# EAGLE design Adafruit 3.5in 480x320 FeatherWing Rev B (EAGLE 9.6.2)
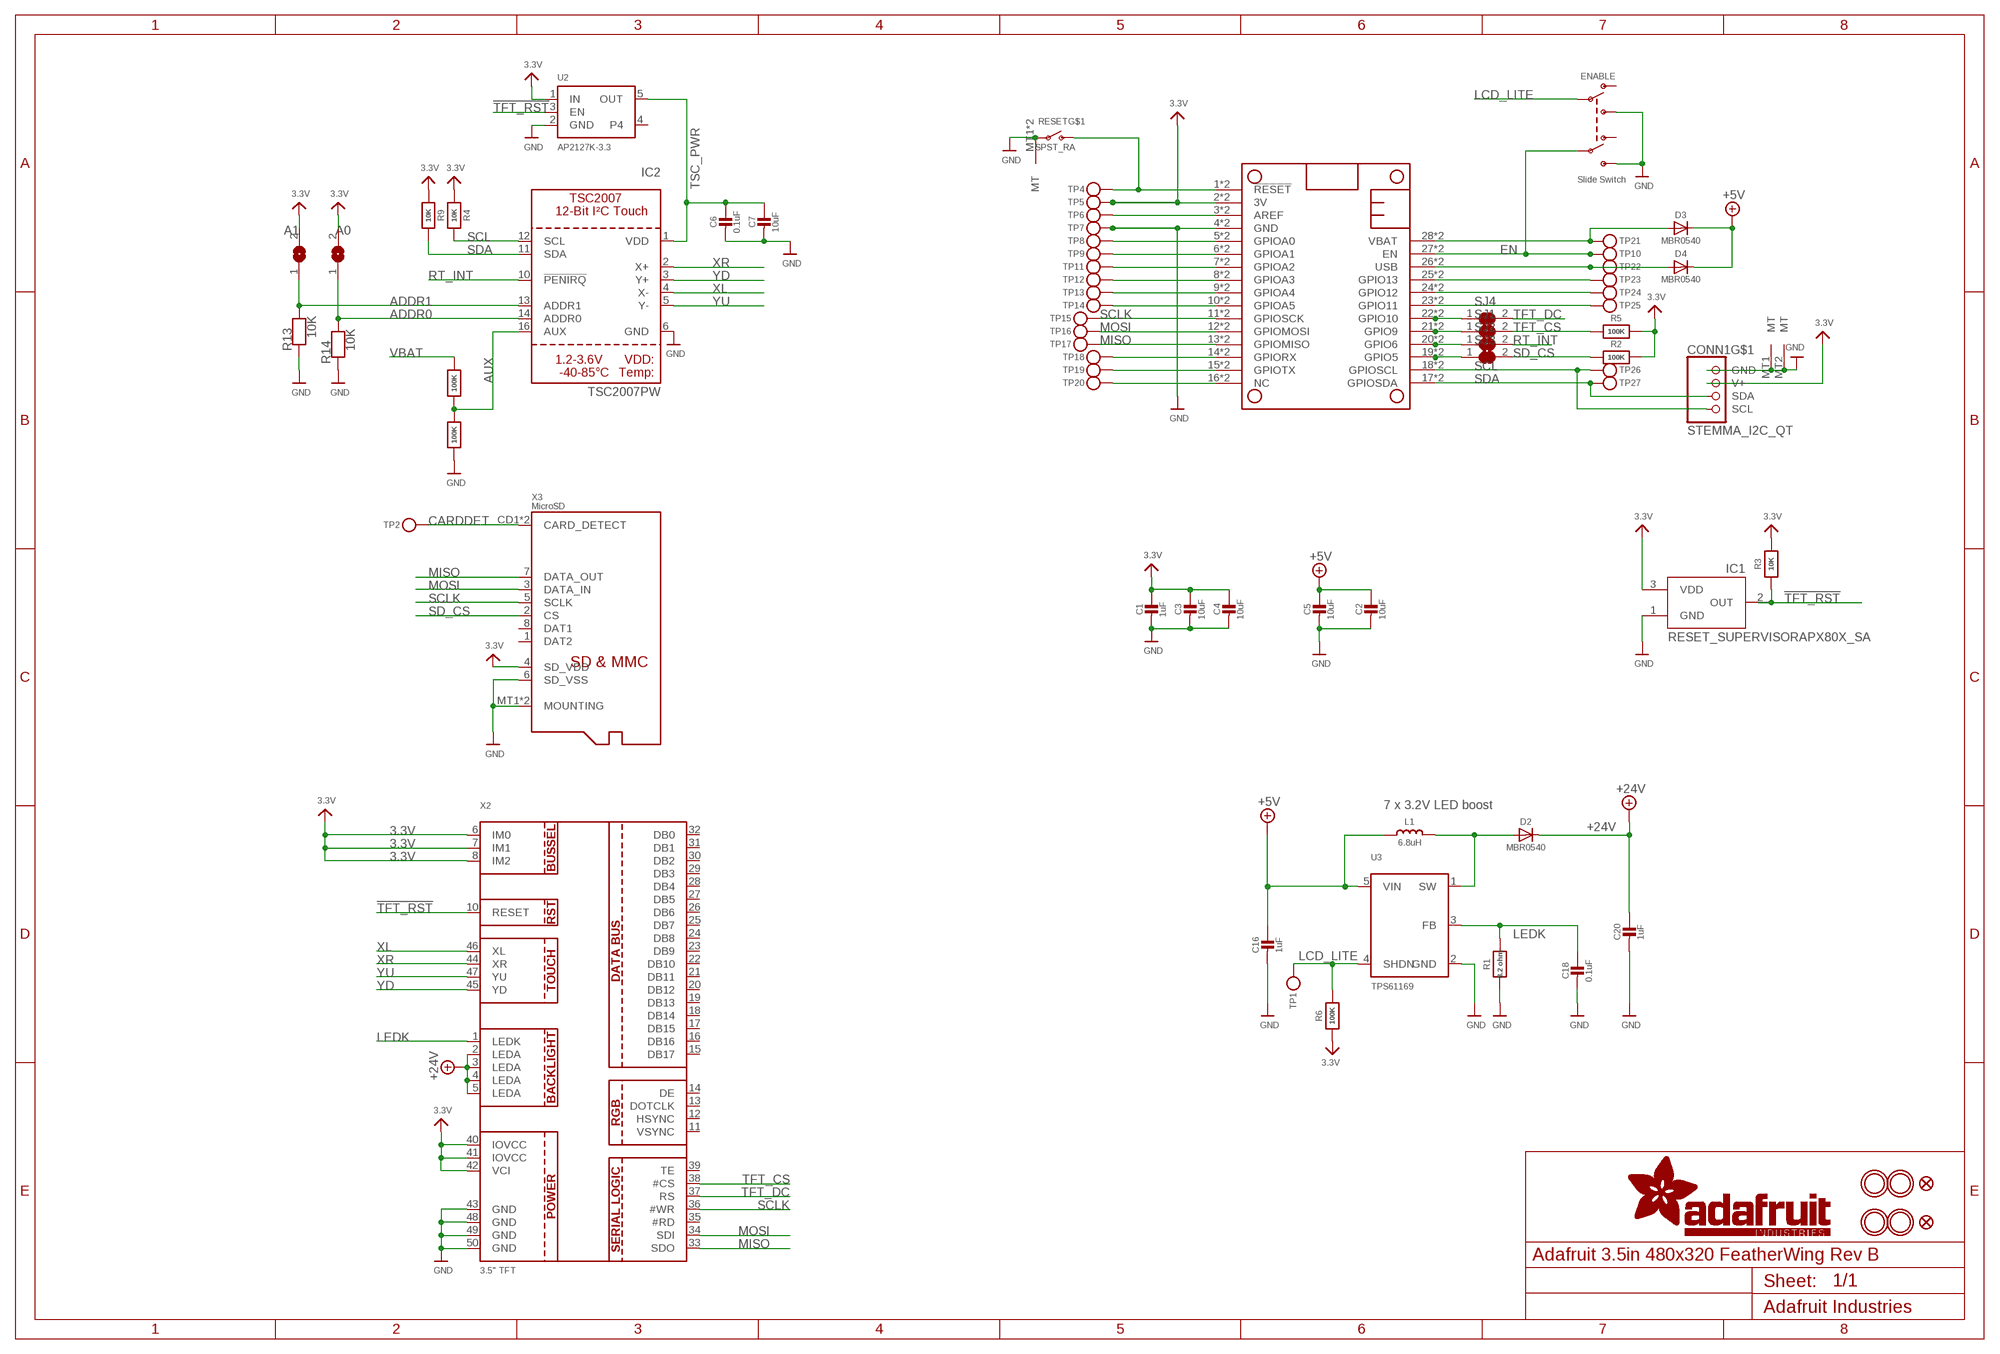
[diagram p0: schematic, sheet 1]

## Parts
C1  1uF  CAP_CERAMIC0805-NOOUTLINE  [0805-NO]
C2  10uF  CAP_CERAMIC0805-NOOUTLINE  [0805-NO]
C3  10uF  CAP_CERAMIC0805-NOOUTLINE  [0805-NO]
C4  10uF  CAP_CERAMIC0805-NOOUTLINE  [0805-NO]
C5  10uF  CAP_CERAMIC0805-NOOUTLINE  [0805-NO]
C6  0.1uF  CAP_CERAMIC0603_NO  [0603-NO]
C7  10uF  CAP_CERAMIC0805-NOOUTLINE  [0805-NO]
C16  1uF  CAP_CERAMIC0805-NOOUTLINE  [0805-NO]
C18  0.1uF  CAP_CERAMIC0603_NO  [0603-NO]
C20  1uF  CAP_CERAMIC0805-NOOUTLINE  [0805-NO]
CONN1  STEMMA_I2C_QT  [JST_SH4]
D2  MBR0540  DIODESOD-123  [SOD-123]
D3  MBR0540  DIODESOD-123  [SOD-123]
D4  MBR0540  DIODESOD-123  [SOD-123]
ENABLE  Slide Switch  SWITCH_DPDTEG1390  [EG1390]
IC1  RESET_SUPERVISORAPX80X_SA  [SOT23-WIDE]
IC2  TSC2007PW  [TSSOP16]
ICSP_CLK1  A1  SOLDERJUMPER  [SOLDERJUMPER_ARROW_NOPASTE]
ICSP_CLK2  A0  SOLDERJUMPER  [SOLDERJUMPER_ARROW_NOPASTE]
L1  6.8uH  INDUCTORNR5040  [INDUCTOR_5X5MM_NR5040_NOTHERMALS]
MS2  FEATHERWING_SMTDUAL  [FEATHERWING_SMT2]
R1  8.2 ohm  RESISTOR_0603_NOOUT  [0603-NO]
R2  100K  RESISTOR_0603_NOOUT  [0603-NO]
R3  10K  RESISTOR_0603_NOOUT  [0603-NO]
R4  10K  RESISTOR_0603_NOOUT  [0603-NO]
R5  100K  RESISTOR_0603_NOOUT  [0603-NO]
R6  100K  RESISTOR_0603_NOOUT  [0603-NO]
R9  10K  RESISTOR_0603_NOOUT  [0603-NO]
R10  100K  RESISTOR_0603_NOOUT  [0603-NO]
R11  100K  RESISTOR_0603_NOOUT  [0603-NO]
R13  10K  RESISTOR_0603_NOOUT  [0603-NO]
R14  10K  RESISTOR_0603_NOOUT  [0603-NO]
RESET  SPST_RA  SWITCH_SPST_MNT_TACT_RA  [SPST_TACTILE_RA]
SJ1  SOLDERJUMPER_CLOSED  [SOLDERJUMPER_CLOSEDWIRE]
SJ2  SOLDERJUMPER_CLOSED  [SOLDERJUMPER_CLOSEDWIRE]
SJ3  SOLDERJUMPER_CLOSED  [SOLDERJUMPER_CLOSEDWIRE]
SJ4  SOLDERJUMPER_CLOSED  [SOLDERJUMPER_CLOSEDWIRE]
TP1  TESTPOINTPAD2MM  [TESTPOINT_PAD_2MM]
TP2  TESTPOINTPAD2MM  [TESTPOINT_PAD_2MM]
TP4  TESTPOINTPAD2MM  [TESTPOINT_PAD_2MM]
TP5  TESTPOINTPAD2MM  [TESTPOINT_PAD_2MM]
TP6  TESTPOINTPAD2MM  [TESTPOINT_PAD_2MM]
TP7  TESTPOINTPAD2MM  [TESTPOINT_PAD_2MM]
TP8  TESTPOINTPAD2MM  [TESTPOINT_PAD_2MM]
TP9  TESTPOINTPAD2MM  [TESTPOINT_PAD_2MM]
TP10  TESTPOINTPAD2MM  [TESTPOINT_PAD_2MM]
TP11  TESTPOINTPAD2MM  [TESTPOINT_PAD_2MM]
TP12  TESTPOINTPAD2MM  [TESTPOINT_PAD_2MM]
TP13  TESTPOINTPAD2MM  [TESTPOINT_PAD_2MM]
TP14  TESTPOINTPAD2MM  [TESTPOINT_PAD_2MM]
TP15  TESTPOINTPAD2MM  [TESTPOINT_PAD_2MM]
TP16  TESTPOINTPAD2MM  [TESTPOINT_PAD_2MM]
TP17  TESTPOINTPAD2MM  [TESTPOINT_PAD_2MM]
TP18  TESTPOINTPAD2MM  [TESTPOINT_PAD_2MM]
TP19  TESTPOINTPAD2MM  [TESTPOINT_PAD_2MM]
TP20  TESTPOINTPAD2MM  [TESTPOINT_PAD_2MM]
TP21  TESTPOINTPAD2MM  [TESTPOINT_PAD_2MM]
TP22  TESTPOINTPAD2MM  [TESTPOINT_PAD_2MM]
TP23  TESTPOINTPAD2MM  [TESTPOINT_PAD_2MM]
TP24  TESTPOINTPAD2MM  [TESTPOINT_PAD_2MM]
TP25  TESTPOINTPAD2MM  [TESTPOINT_PAD_2MM]
TP26  TESTPOINTPAD2MM  [TESTPOINT_PAD_2MM]
TP27  TESTPOINTPAD2MM  [TESTPOINT_PAD_2MM]
U2  AP2127K-3.3  VREG_SOT23-5  [SOT23-5]
U3  TPS61169  VREG_BOOST_5PIN_SC70  [SC70-5]
U$7  MOUNTINGHOLE3.0THIN  [MOUNTINGHOLE_3.0_PLATEDTHIN]
U$9  FIDUCIAL_1MM  [FIDUCIAL_1MM]
U$15  MOUNTINGHOLE3.0THIN  [MOUNTINGHOLE_3.0_PLATEDTHIN]
U$16  MOUNTINGHOLE3.0THIN  [MOUNTINGHOLE_3.0_PLATEDTHIN]
U$17  MOUNTINGHOLE3.0THIN  [MOUNTINGHOLE_3.0_PLATEDTHIN]
U$23  FIDUCIAL_1MM  [FIDUCIAL_1MM]
X2  3.5" TFT  DISP_LCD_3.5IN_320X480_50PIN  [TFT_3.5IN_320X480_50PIN]
X3  MicroSD  MICROSD  [MICROSD]

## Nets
3.3V: C1.1 C3.1 C4.1 CONN1.2(V+) IC1.3(VDD) ICSP_CLK1.2 ICSP_CLK2.2 MS2.2'(3V) MS2.2(3V) R2.2 R3.2 R4.1 R5.2 R6.1 R9.1 TP5.P$1 U2.1(IN) X2.6(IM0) X2.7(IM1) X2.8(IM2) X2.40(IOVCC) X2.41(IOVCC) X2.42(VCI) X3.4(SD_VDD)
!RESET: MS2.1'(!RESET) MS2.1(!RESET) RESET.2(S) TP4.P$1
!TFT_RST: IC1.2(OUT) R3.1 U2.3(EN) X2.10(RESET)
+5V: C2.1 C5.1 C16.1 D3.C D4.C L1.P$1 U3.5(VIN)
+24V: C20.1 D2.C X2.2(LEDA) X2.3(LEDA) X2.4(LEDA) X2.5(LEDA)
A: MS2.5'(GPIOA0) MS2.5(GPIOA0) TP8.P$1
ADDR0: IC2.14(ADDR0) ICSP_CLK2.1 R14.2
ADDR1: IC2.13(ADDR1) ICSP_CLK1.1 R13.2
AREF: MS2.3'(AREF) MS2.3(AREF) TP6.P$1
AUX: IC2.16(AUX) R10.1 R11.2
B: MS2.6'(GPIOA1) MS2.6(GPIOA1) TP9.P$1
C: MS2.7'(GPIOA2) MS2.7(GPIOA2) TP11.P$1
CARDDET: TP2.P$1 X3.CD1(CARD_DETECT) X3.CD2(CARD_DETECT)
D: MS2.8'(GPIOA3) MS2.8(GPIOA3) TP12.P$1
E: MS2.9'(GPIOA4) MS2.9(GPIOA4) TP13.P$1
EN: ENABLE.P2 MS2.27'(EN) MS2.27(EN) TP10.P$1
F: MS2.10'(GPIOA5) MS2.10(GPIOA5) TP14.P$1
G: MS2.16'(NC) MS2.16(NC) TP20.P$1
GND: C1.2 C2.2 C3.2 C4.2 C5.2 C6.2 C7.2 C16.2 C18.2 C20.2 CONN1.1(GND) CONN1.MT1(MT) CONN1.MT2(MT) ENABLE.S1 ENABLE.S2 IC1.1(GND) IC2.6(GND) MS2.4'(GND) MS2.4(GND) R1.1 R11.1 R13.1 R14.1 RESET.1(P) RESET.MT1(MT) RESET.MT2(MT) TP7.P$1 U2.2(GND) U3.2(GND) X2.43(GND) X2.48(GND) X2.49(GND) X2.50(GND) X3.6(SD_VSS) X3.MT1(MOUNTING) X3.MT2(MOUNTING)
H: MS2.19'(GPIO5) MS2.19(GPIO5) SJ3.1
I: MS2.20'(GPIO6) MS2.20(GPIO6) SJ2.1
J: MS2.21'(GPIO9) MS2.21(GPIO9) SJ1.1
K: MS2.22'(GPIO10) MS2.22(GPIO10) SJ4.1
L: MS2.23'(GPIO11) MS2.23(GPIO11) TP25.P$1
LCD_LITE: ENABLE.P1 R6.2 TP1.P$1 U3.4(SHDN)
LEDK: C18.1 R1.2 U3.3(FB) X2.1(LEDK)
M: MS2.24'(GPIO12) MS2.24(GPIO12) TP24.P$1
MISO: MS2.13'(GPIOMISO) MS2.13(GPIOMISO) TP17.P$1 X2.33(SDO) X3.7(DATA_OUT)
MOSI: MS2.12'(GPIOMOSI) MS2.12(GPIOMOSI) TP16.P$1 X2.34(SDI) X3.3(DATA_IN)
N: MS2.25'(GPIO13) MS2.25(GPIO13) TP23.P$1
N$3: D2.A L1.P$2 U3.1(SW)
RT_INT: IC2.10(!PENIRQ) SJ2.2
RX: MS2.14'(GPIORX) MS2.14(GPIORX) TP18.P$1
SCL: CONN1.4(SCL) IC2.12(SCL) MS2.18'(GPIOSCL) MS2.18(GPIOSCL) R4.2 TP26.P$1
SCLK: MS2.11'(GPIOSCK) MS2.11(GPIOSCK) TP15.P$1 X2.36(#WR) X3.5(SCLK)
SD_CS: R2.1 SJ3.2 X3.2(CS)
SDA: CONN1.3(SDA) IC2.11(SDA) MS2.17'(GPIOSDA) MS2.17(GPIOSDA) R9.2 TP27.P$1
TFT_CS: R5.1 SJ1.2 X2.38(#CS)
TFT_DC: SJ4.2 X2.37(RS)
TSC_PWR: C6.1 C7.1 IC2.1(VDD) U2.5(OUT)
TX: MS2.15'(GPIOTX) MS2.15(GPIOTX) TP19.P$1
USB: D4.A MS2.26'(USB) MS2.26(USB) TP22.P$1
VBAT: D3.A MS2.28'(VBAT) MS2.28(VBAT) R10.2 TP21.P$1
XL: IC2.4(X-) X2.46(XL)
XR: IC2.2(X+) X2.44(XR)
YD: IC2.3(Y+) X2.45(YD)
YU: IC2.5(Y-) X2.47(YU)
Unconnected: ENABLE.O1 ENABLE.O2 U2.4 X2.11(VSYNC) X2.12(HSYNC) X2.13(DOTCLK) X2.14(DE) X2.15(DB17) X2.16(DB16) X2.17(DB15) X2.18(DB14) X2.19(DB13) X2.20(DB12) X2.21(DB11) X2.22(DB10) X2.23(DB9) X2.24(DB8) X2.25(DB7) X2.26(DB6) X2.27(DB5) X2.28(DB4) X2.29(DB3) X2.30(DB2) X2.31(DB1) X2.32(DB0) X2.35(#RD) X2.39(TE) X3.1(DAT2) X3.8(DAT1)

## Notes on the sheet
- 7 x 3.2V LED boost

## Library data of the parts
C1-C7 C16 C18 C20 = microbuilder:CAP_CERAMIC: Ceramic Capacitors
CONN1 = adafruit_electromech:STEMMA_I2C; LCSC: C2845363
D2-D4 = microbuilder:DIODE: Diode
ENABLE = adafruit_electromech:SWITCH_DPDT: Switch - DPDT A DPDT Switch acts like an SPDT switch, but has a pair of switches instead of just one. Vertical - 0.3A @ 6V SMT - Digikey: JS202011SCQN; LCSC: C2837066
IC1 = adafruit_power:RESET_SUPERVISOR; ROT: 270
IC2 = adafruit_sensor:TSC2007
ICSP_CLK1 ICSP_CLK2 = microbuilder:SOLDERJUMPER: SMD Solder JUMPER; BOM: EXCLUDE
L1 = microbuilder:INDUCTOR: Inductors
MS2 = microbuilder:FEATHERWING
R1-R6 R9-R11 R13 R14 = microbuilder:RESISTOR: Resistors
RESET = adafruit_electromech:SWITCH_SPST_MNT: Switch - SPST 4UCon 19192 (6.7x2.6mm SMT); LCSC: C778159
SJ1-SJ4 = microbuilder:SOLDERJUMPER_CLOSED: Solder Jumper - Closed
TP1 TP2 TP4-TP27 = microbuilder:TESTPOINT: Test Point
U2 = adafruit_power:VREG_SOT23-5: SOT23-5 Fixed Voltage Regulators Part Current Out V Out V In V Dropout θJA (°C/W) TJ (°C) Digikey Part No. ADP121 150mA 3.3V 3.4-5.5V 0.09V @ 150mA -- -- ADP121-AUJZ33R7CT-ND ADP121 150mA 3.0V 3.1-5.5V 0.09V @ 150mA -- -- ADP121-AUJZ30R7CT-ND ADP122 300mA 3.3V 3.4-5.5V 0.085V @ 300mA -- --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; JLC_ROTATION: 270
U3 = adafruit_power:VREG_BOOST_5PIN: FAN5331 - LED/OLED 20V Boost Converter Digikey: FAN5331SXCT-ND
U$7 U$15-U$17 = adafruit_electromech:MOUNTINGHOLE: Mounting Hole; BOM: EXCLUDE
U$9 U$23 = microbuilder:FIDUCIAL: Fiducial Alignment Points; BOM: EXCLUDE
X2 = adafruit_display:DISP_LCD_3.5IN_320X480_50PIN: DT350HV15-T - 3.5" 320x480 TFT Display, 50 Pin Connector
X3 = adafruit_electromech:MICROSD: MicroSD/Transflash Card Holder with SPI pinout 3M: 2908-05WB-MG 4UConnector: 19656 Footprint courtesy: Adafruit Industries; JLC_ROTATION: 90; LCSC: C125617

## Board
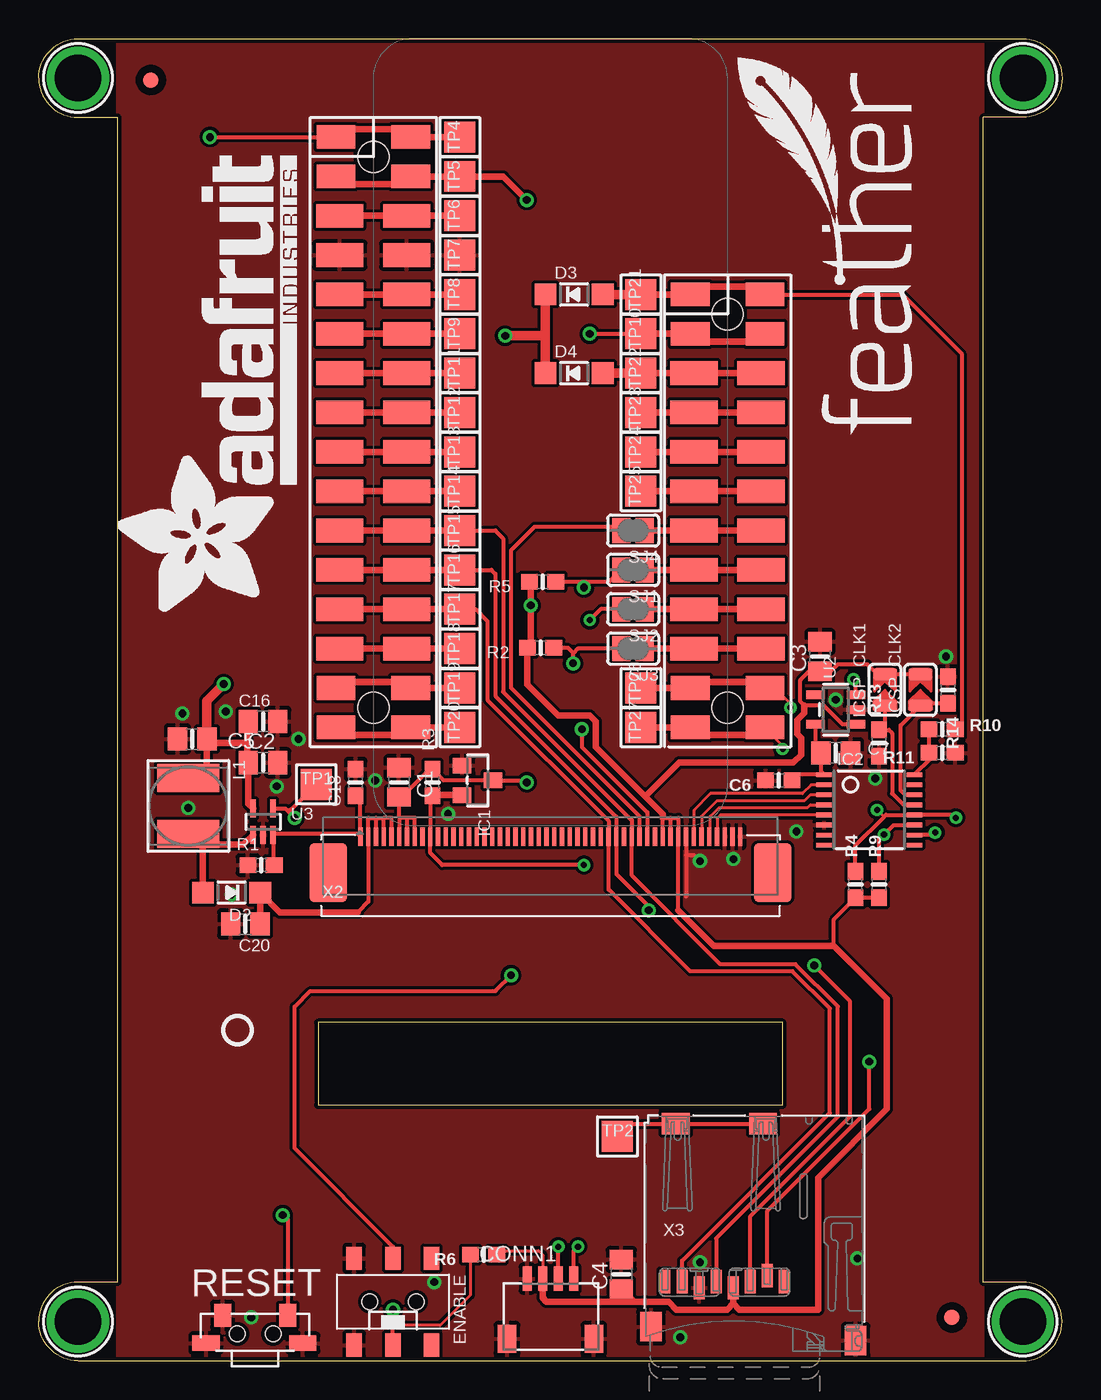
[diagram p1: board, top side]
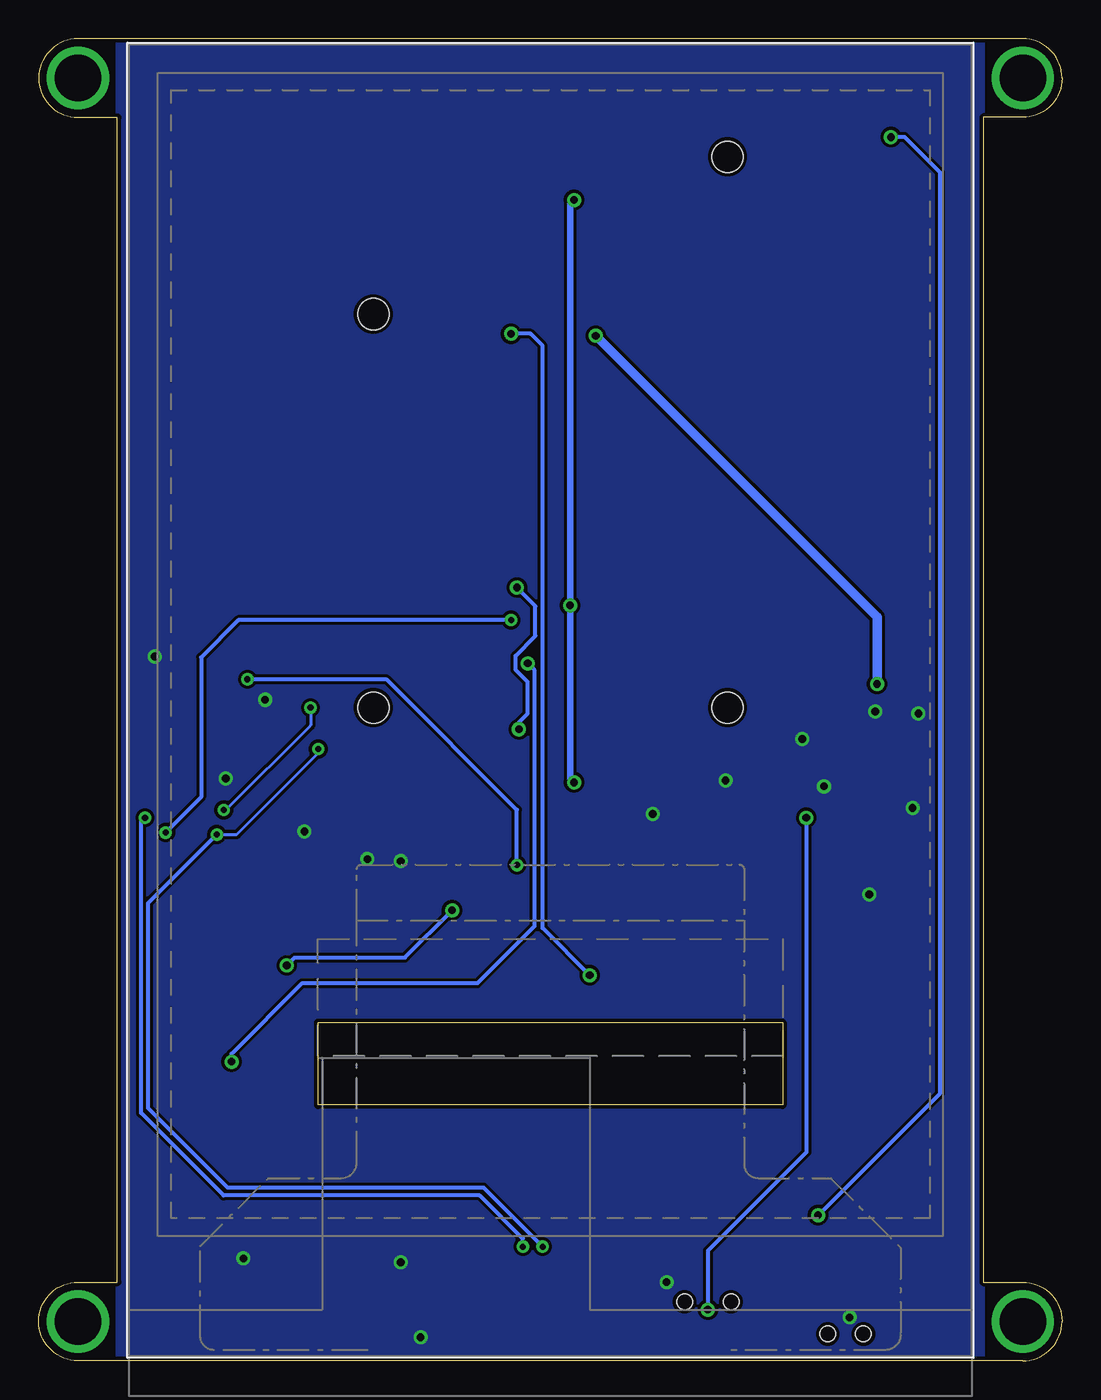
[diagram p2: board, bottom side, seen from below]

Size 66.04 x 85.34 mm. Coordinates in mm from the lower left corner, seen from the top.
Outline: 2.54,0 63.5,0 arc90 66.04,2.54 arc90 63.5,5.08 60.96,5.08 60.96,80.26 63.5,80.26 arc90 66.04,82.8 arc90 63.5,85.34 2.54,85.34 arc90 0,82.8 arc90 2.54,80.26 5.08,80.26 5.08,5.08 2.54,5.08 arc90 0,2.54 arc90 2.54,0
Outline: 18.03,21.84 18.03,16.51 48.01,16.51 48.01,21.84 18.03,21.84
Copper layers (1*16): Top 0.035mm / dielectric 1.5mm / Bottom 0.035mm
Design rules "adafruit *": minimum track width 8mil, minimum drill 15.5mil, track to track 8mil, track to pad 8mil, pad to pad 8mil, via to via 8mil, smd to smd 8mil, copper to edge 10mil, drill to drill 8mil, minimum pad ring 10mil, minimum via ring 8mil, stop-mask expansion 2mil, vias tented up to drill 20mil, thermal gap 10mil
tRestrict: area 44.5,33.7 to 44.6,34; area 45,33.7 to 45.1,34

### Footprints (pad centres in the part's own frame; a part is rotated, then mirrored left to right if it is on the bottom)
0805-NO = smd 1.24 x 1.5: 1 -0.95,0; 2 0.95,0
0603-NO = smd 1.075 x 1: 1 -0.85,0; 2 0.85,0
JST_SH4 = smd 0.6 x 1.55: 1 -1.5,2.006; 2 -0.5,2.006; 3 0.5,2.006; 4 1.5,2.006 | smd 1.2 x 1.8: MT1 -2.8,-1.894; MT2 2.8,-1.894
SOD-123 = smd 1.4 x 1.4: A 1.85,0; C -1.85,0
EG1390 = smd 1 x 1.5: O1 -2.5,2.8; O2 -2.5,-2.8; P1 0,2.8; P2 0,-2.8; S1 2.5,2.8; S2 2.5,-2.8 | hole 1: 1.5,0; -1.5,0
SOT23-WIDE = smd 1 x 1.2: 1 -0.95,-1; 2 0.95,-1; 3 0,1
TSSOP16 = smd 0.305 x 0.991: 1 -2.275,-2.918; 2 -1.625,-2.918; 3 -0.975,-2.918; 4 -0.325,-2.918; 5 0.325,-2.918; 6 0.975,-2.918; 7 1.625,-2.918; 8 2.275,-2.918; 9 2.275,2.918; 10 1.625,2.918; 11 0.975,2.918; 12 0.325,2.918; 13 -0.325,2.918; 14 -0.975,2.918; 15 -1.625,2.918; 16 -2.275,2.918
SOLDERJUMPER_ARROW_NOPASTE = smd 0.762 x 1.524: 1 -1.016,0; 2 1.016,0
INDUCTOR_5X5MM_NR5040_NOTHERMALS = smd 1.8 x 4: P$1 -1.8,0; P$2 1.8,0
FEATHERWING_SMT2 = smd 1.524 x 2.5: 1 6.35,2.413; 1' 6.35,-2.413; 2 8.89,2.413; 2' 8.89,-2.413; 15 41.91,2.413; 15' 41.91,-2.413; 16 44.45,2.413; 16' 44.45,-2.413; 17 44.45,20.447; 17' 44.45,25.273; 18 41.91,20.447; 18' 41.91,25.273; 27 19.05,20.447; 27' 19.05,25.273; 28 16.51,20.447; 28' 16.51,25.273 | smd 1.524 x 3.048: 3 11.43,2.159; 3' 11.43,-2.159; 4 13.97,2.159; 4' 13.97,-2.159; 5 16.51,2.159; 5' 16.51,-2.159; 6 19.05,2.159; 6' 19.05,-2.159; 7 21.59,2.159; 7' 21.59,-2.159; 8 24.13,2.159; 8' 24.13,-2.159; 9 26.67,2.159; 9' 26.67,-2.159; 10 29.21,2.159; 10' 29.21,-2.159; 11 31.75,2.159; 11' 31.75,-2.159; 12 34.29,2.159; 12' 34.29,-2.159; 13 36.83,2.159; 13' 36.83,-2.159; 14 39.37,2.159; 14' 39.37,-2.159; 19 39.37,20.701; 19' 39.37,25.019; 20 36.83,20.701; 20' 36.83,25.019; 21 34.29,20.701; 21' 34.29,25.019; 22 31.75,20.701; 22' 31.75,25.019; 23 29.21,20.701; 23' 29.21,25.019; 24 26.67,20.701; 24' 26.67,25.019; 25 24.13,20.701; 25' 24.13,25.019; 26 21.59,20.701; 26' 21.59,25.019 | hole 2: 17.78,22.86; 43.18,22.86; 7.62,0; 43.18,0
SPST_TACTILE_RA = smd 1.1 x 1.5: 1 2.1,-0.9; 2 -2.1,-0.9 | smd 1.75 x 1: MT1 3.175,0.9; MT2 -3.075,0.9 | hole 1: 1.15,0.3; -1.15,0.3
SOLDERJUMPER_CLOSEDWIRE = smd 1.168 x 1.6: 1 -0.762,0; 2 0.762,0 | smd 0.635 x 0.203: WIRE 0,0
TESTPOINT_PAD_2MM = smd 2 x 2: P$1 0,0
SOT23-5 = smd 0.55 x 1.2: 1 -0.95,-1.3; 2 0,-1.3; 3 0.95,-1.3; 4 0.95,1.3; 5 -0.95,1.3
SC70-5 = smd 0.35 x 1.15: 1 -0.65,-0.85; 2 0,-0.85; 3 0.65,-0.85; 4 0.65,0.85; 5 -0.65,0.85
MOUNTINGHOLE_3.0_PLATEDTHIN = drill 3 pad 3.6: P$1 0,0
FIDUCIAL_1MM = smd 1 x 1: 1 0,0
TFT_3.5IN_320X480_50PIN = smd 0.275 x 1.2 bottom: 1 12.25,1.066; 2 11.75,1.066; 3 11.25,1.066; 4 10.75,1.066; 5 10.25,1.066; 6 9.75,1.066; 7 9.25,1.066; 8 8.75,1.066; 9 8.25,1.066; 10 7.75,1.066; 11 7.25,1.066; 12 6.75,1.066; 13 6.25,1.066; 14 5.75,1.066; 15 5.25,1.066; 16 4.75,1.066; 17 4.25,1.066; 18 3.75,1.066; 19 3.25,1.066; 20 2.75,1.066; 21 2.25,1.066; 22 1.75,1.066; 23 1.25,1.066; 24 0.75,1.066; 25 0.25,1.066; 26 -0.25,1.066; 27 -0.75,1.066; 28 -1.25,1.066; 29 -1.75,1.066; 30 -2.25,1.066; 31 -2.75,1.066; 32 -3.25,1.066; 33 -3.75,1.066; 34 -4.25,1.066; 35 -4.75,1.066; 36 -5.25,1.066; 37 -5.75,1.066; 38 -6.25,1.066; 39 -6.75,1.066; 40 -7.25,1.066; 41 -7.75,1.066; 42 -8.25,1.066; 43 -8.75,1.066; 44 -9.25,1.066; 45 -9.75,1.066; 46 -10.25,1.066; 47 -10.75,1.066; 48 -11.25,1.066; 49 -11.75,1.066; 50 -12.25,1.066 | smd 2.4 x 3.81 bottom: PAD1 14.35,-1.253; PAD2 -14.35,-1.253
MICROSD = smd 0.7 x 1.5: 1 1.761,-3.147; 2 0.661,-2.747; 3 -0.439,-3.147; 4 -1.539,-3.547; 5 -2.639,-3.147; 6 -3.739,-3.547; 7 -4.839,-3.147; 8 -5.939,-3.147 | smd 1.8 x 1.4: CD1 -5.239,7.053; CD2 0.38,7.053 | smd 1.4 x 1.9: MT1 -6.839,-6.047; MT2 6.361,-6.947

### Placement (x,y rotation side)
C1  23.24,37.34 90 top
C2  14.48,38.61 0 top
C3  50.42,45.47 90 top
C4  37.59,5.59 90 top
C5  9.91,40.13 180 top
C6  47.75,37.46 180 top
C7  51.44,39.24 0 top
C16  14.48,41.27 0 top
C18  20.45,37.34 90 top
C20  13.34,28.19 180 top
CONN1  33.02,3.3 0 top
D2  12.45,30.23 180 top
D3  34.54,68.83 0 top
D4  34.54,63.75 0 top
ENABLE  22.86,3.81 180 top
IC1  28.32,37.46 270 top
IC2  53.59,35.56 270 top
ICSP_CLK1  54.61,43.31 90 top
ICSP_CLK2  56.9,43.31 90 top
L1  9.65,35.81 270 top
MS2  21.59,85.34 270 top
PLABEL0  [PLABEL0]  28.19,2.92 90 top
PLABEL1  [PLABEL1]  18.92,2.67 90 top
PLABEL2  [PLABEL2]  11.3,3.94 0 top
PLABEL3  [PLABEL3]  19.81,7.87 0 top
PLABEL4  [PLABEL4]  17.27,34.54 0 top
PLABEL5  [PLABEL5]  36.45,53.59 0 top
PLABEL6  [PLABEL6]  36.45,51.05 0 top
PLABEL7  [PLABEL7]  36.45,48.64 0 top
PLABEL8  [PLABEL8]  36.45,45.97 0 top
PLABEL9  [PLABEL9]  8.64,17.78 90 top
PLABEL10  [PLABEL10]  57.4,45.47 90 top
PLABEL11  [PLABEL11]  55.12,45.47 90 top
PLABEL12  [PLABEL12]  38.73,12.19 0 top
PLABEL13  [PLABEL13]  59.69,14.48 90 top
PLABEL14  [PLABEL14]  55.63,0.76 90 top
PLABEL15  [PLABEL15]  30.23,6.6 0 top
R1  14.35,32 0 top
R2  32.39,46.04 180 top
R3  25.4,37.34 90 top
R4  52.7,30.73 90 top
R5  32.51,50.29 180 top
R6  28.7,6.86 180 top
R9  54.23,30.73 90 top
R10  58.29,40.77 0 top
R11  58.29,39.24 180 top
R13  54.23,39.88 90 top
R14  58.67,43.31 270 top
RESET  13.97,2.03 180 top
SJ1  38.35,51.05 180 top
SJ2  38.35,48.51 180 top
SJ3  38.35,45.97 180 top
SJ4  38.35,53.59 180 top
TP1  17.91,37.21 0 top
TP2  37.34,14.48 0 top
TP4  27.18,78.99 90 top
TP5  27.18,76.45 90 top
TP6  27.18,73.91 90 top
TP7  27.18,71.37 90 top
TP8  27.18,68.83 90 top
TP9  27.18,66.29 90 top
TP10  38.86,66.29 90 top
TP11  27.18,63.75 90 top
TP12  27.18,61.21 90 top
TP13  27.18,58.67 90 top
TP14  27.18,56.13 90 top
TP15  27.18,53.59 90 top
TP16  27.18,51.05 90 top
TP17  27.18,48.51 90 top
TP18  27.18,45.97 90 top
TP19  27.18,43.43 90 top
TP20  27.18,40.89 90 top
TP21  38.86,68.83 90 top
TP22  38.86,63.75 90 top
TP23  38.86,61.21 90 top
TP24  38.86,58.67 90 top
TP25  38.86,56.13 90 top
TP26  38.86,43.43 90 top
TP27  38.86,40.89 90 top
U2  51.44,42.04 90 top
U3  14.48,34.8 0 top
U$7  2.54,2.54 0 top
U$9  58.93,2.79 0 top
U$11  [FEATHERLOGO]  56.39,59.82 90 top
U$15  63.5,2.54 0 top
U$16  2.54,82.8 0 top
U$17  63.5,82.8 0 top
U$19  [ADAFRUIT_TEXT_30MM]  16.64,48.13 90 top
U$23  7.24,82.68 0 top
U$37  [PCBFEAT-REV-040]  12.83,21.34 90 top
X2  33.02,32.77 0 bottom
X3  46.36,8.25 0 top

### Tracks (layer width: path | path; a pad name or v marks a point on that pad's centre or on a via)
3.3V  (via drill 0.5)
  Top 0.203: R6.1 29.81,7.11 32.26,7.11 32.52,6.85 CONN1.2
  Top 0.254: 23.77,35.05 23.27,35.05 | X2.8 24.27,35.05 23.77,35.05 | X2.7 23.77,35.05 | 23.27,35.05 23.27,36.39 C1.1 23.43,36.39 25.23,38.19 R3.2 26.12,37.46 IC1.3 31.37,37.46 v31.5,37.34 | 40.77,35.05 40.27,35.05 X2.40 | X2.41 40.77,35.05 | 41.27,29.09 X2.42 41.27,35.05 40.77,35.05 | 23.27,35.05 X2.6 | ICSP_CLK2.2 ICSP_CLK1.2 54.1,44.32 53.47,44.96 51.56,44.96 51.12,44.52 C3.1 49.72,44.52 49.15,43.94 49.15,42.55 49.4,42.29 50.67,42.29 51.88,41.09 U2.1 | R9.1 R4.1 51.31,28.49 51.31,26.8
  Top 0.406: X3.4 44.82,3.7 | 44.82,3.7 45.21,3.3 50.29,3.3 50.29,11.81 54.74,16.26 54.74,23.37 51.31,26.8 43.56,26.8 41.27,29.09 | 38.42,3.81 40.64,3.81 41.15,3.3 44.42,3.3 44.82,3.7 | C4.1 38.42,3.81 | v31.5,74.93 29.97,76.45 TP5.P$1 MS2.2 23.88,76.45 23.37,75.95 19.69,75.95 MS2.2' | 40.27,35.05 40.27,35.3 39.15,36.42 | 39.15,36.42 35.94,39.62 35.94,41.27 35.56,41.66 33.53,41.66 31.54,43.65 R2.2 31.75,46.25 v31.75,48.77 31.75,50.2 R5.2 | 39.15,36.42 41.34,38.61 48.7,38.61 49.21,39.12 49.21,40.2 48.96,40.45 48.96,41.36 49.4,41.8 49.4,42.29 | CONN1.2 32.52,4.06 32.77,3.81 38.42,3.81
  Bottom 0.254: v31.5,37.34 31.75,37.59 | 31.75,48.01 v31.75,48.77
  Bottom 0.406: 31.75,37.59 31.75,48.01 31.75,74.68 v31.5,74.93
!RESET  (via drill 0.5)
  Top 0.254: v11.05,78.99 MS2.1' | v15.75,9.4 16.07,9.08 RESET.2
  Top 0.406: TP4.P$1 MS2.1 23.75,78.99 23.24,79.5 19.69,79.5 MS2.1'
  Bottom 0.254: v15.75,9.4 7.87,17.27 7.87,76.71 10.16,78.99 v11.05,78.99
!TFT_RST  (via drill 0.39)
  Top 0.254: 25.26,36.24 25.26,33.84 X2.10 25.27,32.77 26.04,32 v35.18,32 | U2.3 52.73,43.84 v52.58,44
  Top 0.406: 25.26,36.24 25.4,36.39 R3.1 25.43,36.52 IC1.2
  Bottom 0.254: v52.58,44 43.62,44 35.18,35.56 v35.18,32
+5V  (via drill 0.5)
  Top 0.406: 13.46,39.88 13.46,38.61 C2.1 13.53,35.95 U3.5 | L1.P$1 10.86,37.61 C5.1 10.86,39.88 13.46,39.88 | 13.46,39.88 13.46,41.21 C16.1
  Top 0.61: D4.C 32.69,66.17 | 32.69,66.17 D3.C | 32.69,66.17 v30.1,66.17 | v11.94,43.69 10.86,42.61 C5.1
  Bottom 0.61: v30.1,66.17 11.94,48.01 v11.94,43.69
+24V
  Top 0.254: 21.77,35.05 21.27,35.05 X2.2 21.27,29.65 20.57,28.96 | 21.77,35.05 22.27,35.05 | X2.5 22.77,35.05 22.27,35.05 | X2.4 22.27,35.05 | X2.3 21.77,35.05
  Top 0.406: 20.57,28.96 15.57,28.96 D2.C 14.3,28.2 C20.1
A
  Top 0.406: TP8.P$1 MS2.5 MS2.5'
ADDR0
  Top 0.254: IC2.14 55.92,36.53 55.63,36.83 55.63,41.02 ICSP_CLK2.1 57.06,42.46 R14.2
ADDR1
  Top 0.254: IC2.13 55.81,35.88 55.07,36.62 55.07,40.52 54.86,40.73 R13.2 54.61,41.11 ICSP_CLK1.1
AREF
  Top 0.406: MS2.3' MS2.3 TP6.P$1
AUX
  Top 0.254: R10.1 R11.2 57.57,39.12 57.57,38.89 IC2.16
B
  Top 0.406: MS2.6' MS2.6 TP9.P$1
C
  Top 0.406: TP11.P$1 MS2.7 MS2.7'
CARDDET
  Top 0.254: X3.CD2 X3.CD1 38.17,15.31 TP2.P$1
D
  Top 0.406: MS2.8' MS2.8 TP12.P$1
E
  Top 0.406: TP13.P$1 MS2.9 MS2.9'
EN  (via drill 0.5)
  Top 0.254: ENABLE.P2 22.86,7.37 16.51,13.72 16.51,22.86 17.53,23.88 29.46,23.88 v30.48,24.89 | v35.56,66.29 TP10.P$1
  Top 0.406: TP10.P$1 MS2.27 42.55,65.79 46.48,65.79 46.86,66.17 MS2.27'
  Bottom 0.254: v30.48,24.89 33.53,27.94 33.53,65.53 34.29,66.29 v35.56,66.29
F
  Top 0.406: TP14.P$1 MS2.10 MS2.10'
G
  Top 0.406: TP20.P$1 MS2.16 23.75,40.89 23.24,40.39 19.69,40.39 MS2.16'
GND  (via drill 0.5)
  Top 0.254: 41.77,29.97 X2.43 41.77,32.65 42.28,32.65 v42.67,32.26
  other vias: 44.83,32.38 16.76,40.13 41.4,1.52 52.83,6.6 42.67,6.35 25.53,5.08 13.72,2.79 21.72,37.46 9.65,35.69 15.37,37.08 12.45,30.1 9.27,41.78 12.07,41.91 26.42,35.31 48.9,34.16 51.44,42.67 58.55,45.47 53.98,37.59
  pour Top: 5.08,85.34 5.08,0 60.96,0 60.96,85.34
  pour Bottom: 5.08,85.34 5.08,0 60.96,0 60.96,85.34
H
  Top 0.406: SJ3.1 MS2.19 MS2.19'
I
  Top 0.406: MS2.20' MS2.20 SJ2.1
J
  Top 0.406: SJ1.1 MS2.21 MS2.21'
K
  Top 0.406: MS2.22' MS2.22 SJ4.1
L
  Top 0.406: TP25.P$1 41.4,56.13 41.4,56.39 42.29,56.39 MS2.23 MS2.23'
LCD_LITE  (via drill 0.5)
  Top 0.203: R6.2 27.85,4.23 25.91,2.29 22.86,2.29
  Top 0.254: U3.4 15.91,35.65 16,35.56 | v16.51,35.05 16,35.56 | ENABLE.P1 22.86,2.29 v22.86,3.3 | 16,35.56 16.26,35.56 TP1.P$1
  Bottom 0.254: v16.51,35.05 16.51,13.46 22.86,7.11 v22.86,3.3
LEDK
  Top 0.254: C18.1 20.45,36.26 20.71,35.99 20.71,33.89 X2.1 20.6,34.01 15.19,34.01 U3.3 15.13,32.08 R1.2
M
  Top 0.406: MS2.24' MS2.24 TP24.P$1
MISO
  Top 0.254: TP17.P$1 28.19,48.51 28.96,47.75 28.96,42.67 36.78,34.85 X2.33 36.77,30.41 42.04,25.15 48.64,25.15 51.05,22.73 51.05,16 41.52,6.46 X3.7
  Top 0.406: TP17.P$1 MS2.13 MS2.13'
MOSI  (via drill 0.5)
  Top 0.254: TP16.P$1 29.21,51.05 29.46,50.8 29.46,42.93 37.27,35.12 X2.34 37.27,31.44 39.37,29.34 v39.37,29.08 | X3.3 45.92,9.34 52.32,15.75 52.32,23.24 v50.04,25.53
  Top 0.406: TP16.P$1 MS2.12 MS2.12'
  Bottom 0.254: v50.04,25.53 49.53,26.03 42.42,26.03 v39.37,29.08
N
  Top 0.406: TP23.P$1 MS2.25 MS2.25'
N$3
  Top 0.406: L1.P$2 10.34,33.32 10.6,33.32 | 10.6,33.32 D2.A | U3.1 13.2,33.32 10.6,33.32
RT_INT  (via drill 0.39)
  Top 0.254: SJ2.2 36.26,48.51 v35.56,47.81 | v57.85,34.1 57.68,33.94 IC2.10
  Bottom 0.254: v35.56,47.81 53.15,47.81 55.56,45.4 55.56,36.39 v57.85,34.1
RX
  Top 0.406: TP18.P$1 MS2.14 MS2.14'
SCL  (via drill 0.39)
  Top 0.203: MS2.18' 47.5,43.43 48.53,42.4 48.53,42.2 v48.5,42.16 | v54.1,35.56 54.55,35.12
  Top 0.254: R4.2 52.7,33.27 54.55,35.12 54.67,35.23 IC2.12 59,35.23 v59.18,35.05 | CONN1.4 34.52,7.09 v34.8,7.37
  Top 0.406: TP26.P$1 MS2.18 42.42,43.81 46.48,43.81 MS2.18'
  Bottom 0.203: v48.5,42.16 48.5,41.02 53.96,35.56 v54.1,35.56
  Bottom 0.254: v34.8,7.37 34.8,7.87 37.59,10.67 54.1,10.67 59.44,16 59.44,34.8 v59.18,35.05
SCLK
  Top 0.254: TP15.P$1 29.46,53.59 29.97,53.09 29.97,43.18 38.27,34.88 X2.36 38.27,31.33 43.99,25.6 48.83,25.6 51.56,22.87 51.56,15.75 43.72,7.9 X3.5
  Top 0.406: TP15.P$1 MS2.11 MS2.11'
SD_CS  (via drill 0.5)
  Top 0.254: X3.2 47.02,9.68 53.59,16.26 v53.59,19.3 | R2.1 34.12,46.04 34.48,45.68 v34.48,45.02 34.48,45.66 34.8,45.97 SJ3.2
  Bottom 0.254: v53.59,19.3 53.59,19.81 49.02,24.38 37.72,24.38 34.04,28.07 34.04,44.58 v34.48,45.02
SDA  (via drill 0.39)
  Top 0.203: v48.01,39.5 48.01,39.69 46.86,40.83 MS2.17'
  Top 0.254: R9.2 54.23,33.66 v54.55,33.97 55.16,34.59 IC2.11 | CONN1.3 v33.52,7.36 v33.53,7.37
  Top 0.406: TP27.P$1 MS2.17 42.55,40.39 46.48,40.39 46.86,40.77 MS2.17'
  Bottom 0.203: v54.55,33.97 53.28,33.97 48.01,39.24 v48.01,39.5
  Bottom 0.254: v33.53,7.37 37.34,11.18 53.85,11.18 58.98,16.31 58.98,29.54 v54.55,33.97
TFT_CS  (via drill 0.5)
  Top 0.254: v35.05,40.77 35.05,39.62 39.27,35.41 X2.38 | R5.1 35.56,50.29 | 35.56,50.29 36.83,50.29 SJ1.2 | 35.56,50.29 v35.18,49.91
  Bottom 0.254: v35.05,40.77 35.05,41.21 34.49,41.77 34.49,43.83 35.26,44.6 35.26,45.51 33.99,46.79 33.99,48.72 v35.18,49.91
TFT_DC
  Top 0.254: X2.37 38.77,35.14 30.48,43.43 30.48,52.32 32,53.85 37.34,53.85 SJ4.2
TSC_PWR
  Top 0.254: C6.1 48.97,37.84 IC2.1 50.48,38.03 C7.1 50.14,39.59 U2.5
TX
  Top 0.406: TP19.P$1 MS2.15 23.75,43.43 23.37,43.81 19.56,43.81 MS2.15'
USB
  Top 0.406: MS2.26' MS2.26 TP22.P$1
  Top 0.61: TP22.P$1 D4.A
VBAT
  Top 0.254: MS2.28' 55.75,68.83 59.56,65.02 59.56,41.19 R10.2
  Top 0.406: TP21.P$1 MS2.28 42.55,69.34 46.23,69.34 46.74,68.83 MS2.28'
  Top 0.61: D3.A TP21.P$1
XL
  Top 0.203: X2.46 43.33,33.89 43.33,35.14 43.88,35.7 49.6,35.7 49.79,35.88 IC2.4
XR
  Top 0.203: IC2.2 49.85,37.19 49.28,36.61 43.34,36.61 42.27,35.54 X2.44
YD
  Top 0.203: IC2.3 49.79,36.53 49.41,36.15 43.77,36.15 42.77,35.16 X2.45
YU
  Top 0.203: IC2.5 44,35.23 43.77,35.01 X2.47

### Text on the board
Pinguin_tBackup: DC | TCS | IRQ | SCS | A1 | A0 | LITE | 3.5" 480x320 TFT / FeatherWing V2 | TSC2007 I2C 0x48 / Touch Controller | SDDET | Stemma / QT I2C | Enable | Reset | OFF | ON | MicroSD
